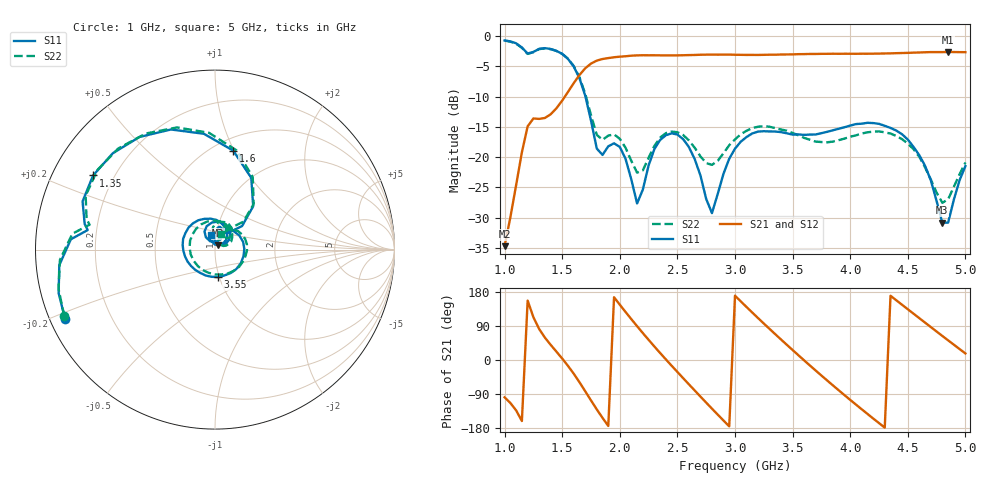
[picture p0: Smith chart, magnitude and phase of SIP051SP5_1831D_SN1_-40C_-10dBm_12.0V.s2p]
# GHz  S  dB  R  50
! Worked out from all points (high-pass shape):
!   81 points, 1 GHz to 5 GHz, reference 50 ohm
!   highest |S21| = -2.63 dB at 4.85 GHz (marker M1); lowest = -34.7 dB at 1 GHz (marker M2)
!   |S21| within 3 dB of the highest: 1.686 GHz to end of sweep
!   lowest |S11| = -30.9 dB at 4.8 GHz (marker M3), VSWR 1.06, Z = 51.5 + j2.51 ohm
!   |S11| at or under -10 dB: 1.702 GHz to end of sweep
!   |S22| runs from -27.6 to -0.7 dB; largest |S21 - S12| = 0.0014
!   S11 on the Smith chart (normalised r, x): 1 GHz: 0.04, -0.22; 1.35 GHz: 0.12, +0.28; 1.6 GHz: 0.62, +0.99; 3.55 GHz: 0.98, -0.31; 5 GHz: 0.94, +0.15
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1  -0.72 -155.1  -34.73 -98.4  -34.84 -98.0  -0.75 -156.2
1.2  -2.88 171.3  -14.92 156.8  -14.90 156.7  -2.94 168.8
1.35  -1.99 148.7  -13.54 59.0  -13.53 58.9  -2.03 145.9
1.6  -5.03 79.6  -7.78 -36.2  -7.76 -36.2  -4.95 77.7
1.7  -9.85 48.6  -5.32 -82.5  -5.33 -82.4  -9.55 49.7
1.8  -18.59 52.1  -4.05 -130.3  -4.06 -130.2  -16.32 53.5
1.95  -17.72 77.9  -3.50 165.6  -3.52 165.6  -16.25 68.4
2.15  -27.67 85.3  -3.19 89.3  -3.19 89.3  -22.57 69.9
2.35  -17.17 109.5  -3.18 18.4  -3.18 18.5  -16.78 89.2
2.5  -16.27 70.8  -3.19 -31.6  -3.18 -31.6  -15.89 60.8
2.7  -23.04 28.8  -3.08 -96.5  -3.08 -96.5  -19.89 40.6
2.8  -29.27 68.5  -3.06 -128.4  -3.04 -128.4  -21.29 53.2
3  -18.61 70.7  -3.08 169.7  -3.08 169.7  -17.08 54.0
3.25  -15.73 1.4  -3.10 96.3  -3.10 96.4  -14.89 9.3
3.55  -16.25 -84.8  -2.99 12.7  -2.98 12.6  -16.40 -60.4
3.7  -16.27 -122.5  -2.95 -27.7  -2.94 -27.7  -17.44 -104.7
4  -14.79 171.8  -2.92 -105.2  -2.93 -105.2  -16.63 160.4
4.35  -15.18 98.2  -2.85 169.5  -2.86 169.5  -16.11 73.1
4.6  -19.69 49.0  -2.71 110.4  -2.70 110.4  -19.96 26.8
4.8  -30.86 58.2  -2.64 63.5  -2.64 63.5  -27.56 37.8
4.85  -30.84 92.6  -2.63 51.9  -2.64 51.9  -26.99 57.4
5  -21.50 106.2  -2.66 17.3  -2.66 17.2  -20.90 69.2
